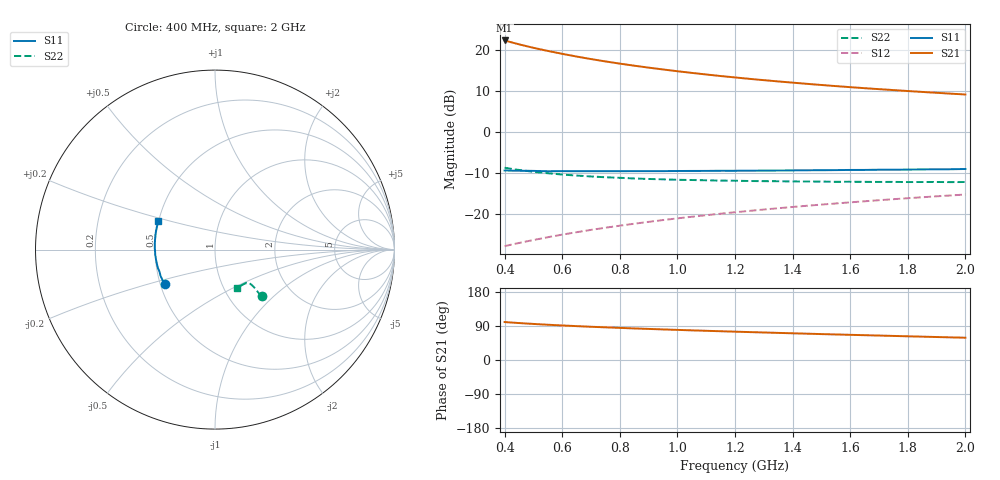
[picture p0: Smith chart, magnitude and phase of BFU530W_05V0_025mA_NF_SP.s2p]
! Filename:  P:\Prog\Test\Noise\ATS_data\Testdata_Net\06 Compressed Noise after Statistics\BFU530W_APM2013_09_A05_05p0V_025mA_NF_CM01_D.sf
! Date/Time: Tue 26/Mar/2013 18:06:04
! BFU530W_APM2013_09_A05_05p0V_1to25mA_NF_CM01_Bias9_R.sf
! Noise Parameter Data File
! BFU530W_APM2013_09_A05_05p0V_1to25mA_NF_CM01
! Date/time: Thu Mar 21 20:31:54 2013
! VAR V_out= 5.001000
! VAR I_out= 25.000000
! VAR V_in= 0.832500
! VAR I_in= 0.269300
! Device data file deembeded for feedlines and parallel
! Original file: \06 Compressed Noise after Statistics\BFU530W_APM2013_09_A05_05p0V_025mA_NF_CM01_R.sf
! Feed-files: PR019V01_070313_Feed1.s2p, PR019V01_070313_Feed2.s2p
! Parallel-file: PR019V01_070313_Par.s2p
# MHz S MA R 50
!  Freq-MHz  S11-mag  S11-arg  S21-mag  S21-arg  S12-mag  S12-arg  S22-mag  S22-arg
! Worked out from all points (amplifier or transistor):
!   37 points, 400 MHz to 2 GHz, reference 50 ohm
!   highest |S21| = 22.2 dB at 400 MHz (marker M1)
!   |S21| within 3 dB of that: start of sweep to 582.3 MHz
!   unconditionally stable (mu >= 1): 878.3 MHz to end of sweep
!   at 500 MHz: K = 0.92, MSG = 23.4 dB, |S12| = -26.3 dB
!   at 1.1 GHz: K = 1.01, MAG = 16.4 dB, |S12| = -20.2 dB
!   at 2 GHz: K = 1.01, MAG = 11.7 dB, |S12| = -15.2 dB
!   lowest NFmin = 1.09 dB at 420 MHz
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400  0.3401 -145.2  12.93 100.2  0.04093 67.8  0.367 -45.0
420  0.3392 -147.5  12.37 99.1  0.04245 68.0  0.3576 -45.0
433  0.3382 -148.9  12.03 98.4  0.04344 68.2  0.3517 -44.9
460  0.3375 -151.2  11.37 97.0  0.04556 68.7  0.3418 -44.8
500  0.3362 -154.9  10.53 95.2  0.04856 69.3  0.3278 -44.5
550  0.3327 -158.5  9.641 93.0  0.05258 70.0  0.3149 -44.2
600  0.334 -161.9  8.891 91.1  0.05653 70.5  0.3034 -44.0
650  0.3334 -165.0  8.241 89.4  0.06049 70.8  0.2951 -43.9
700  0.3332 -167.7  7.679 87.7  0.06455 71.2  0.2878 -43.9
750  0.3334 -170.1  7.191 86.2  0.06854 71.5  0.2814 -43.8
800  0.3332 -172.6  6.761 84.7  0.07262 71.7  0.2771 -44.2
850  0.3342 -174.8  6.381 83.3  0.07668 71.8  0.2719 -44.2
950  0.334 -178.6  5.739 80.7  0.08493 72.1  0.2656 -44.8
1050  0.3358 177.8  5.216 78.2  0.0932 72.1  0.2605 -45.6
1150  0.3375 174.4  4.779 75.9  0.1015 72.0  0.2561 -46.6
1200  0.3374 172.9  4.593 74.8  0.1057 71.9  0.2553 -47.3
1250  0.3383 171.4  4.415 73.7  0.1099 71.8  0.2533 -47.8
1350  0.3397 168.8  4.109 71.5  0.1184 71.5  0.2517 -49.1
1500  0.3426 164.7  3.719 68.4  0.131 70.9  0.2492 -51.5
1600  0.3453 162.1  3.5 66.4  0.1394 70.5  0.2483 -53.1
1750  0.3478 158.6  3.225 63.5  0.1523 69.7  0.2471 -55.5
2000  0.3546 153.0  2.85 58.8  0.1736 68.3  0.2464 -60.3
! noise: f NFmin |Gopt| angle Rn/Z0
400  1.111  0.3201  -172.3  0.0741
460  1.108  0.3283  -170.8  0.0733
600  1.147  0.3259  -166.6  0.0755
800  1.171  0.3327  -163.4  0.0778
1000  1.2  0.3449  -158.8  0.0788
1200  1.235  0.3515  -154.7  0.0848
1400  1.229  0.3613  -150.4  0.0972
1600  1.286  0.3771  -149.6  0.0877
1800  1.312  0.3998  -142.3  0.0967
2000  1.355  0.4206  -137.7  0.1036
